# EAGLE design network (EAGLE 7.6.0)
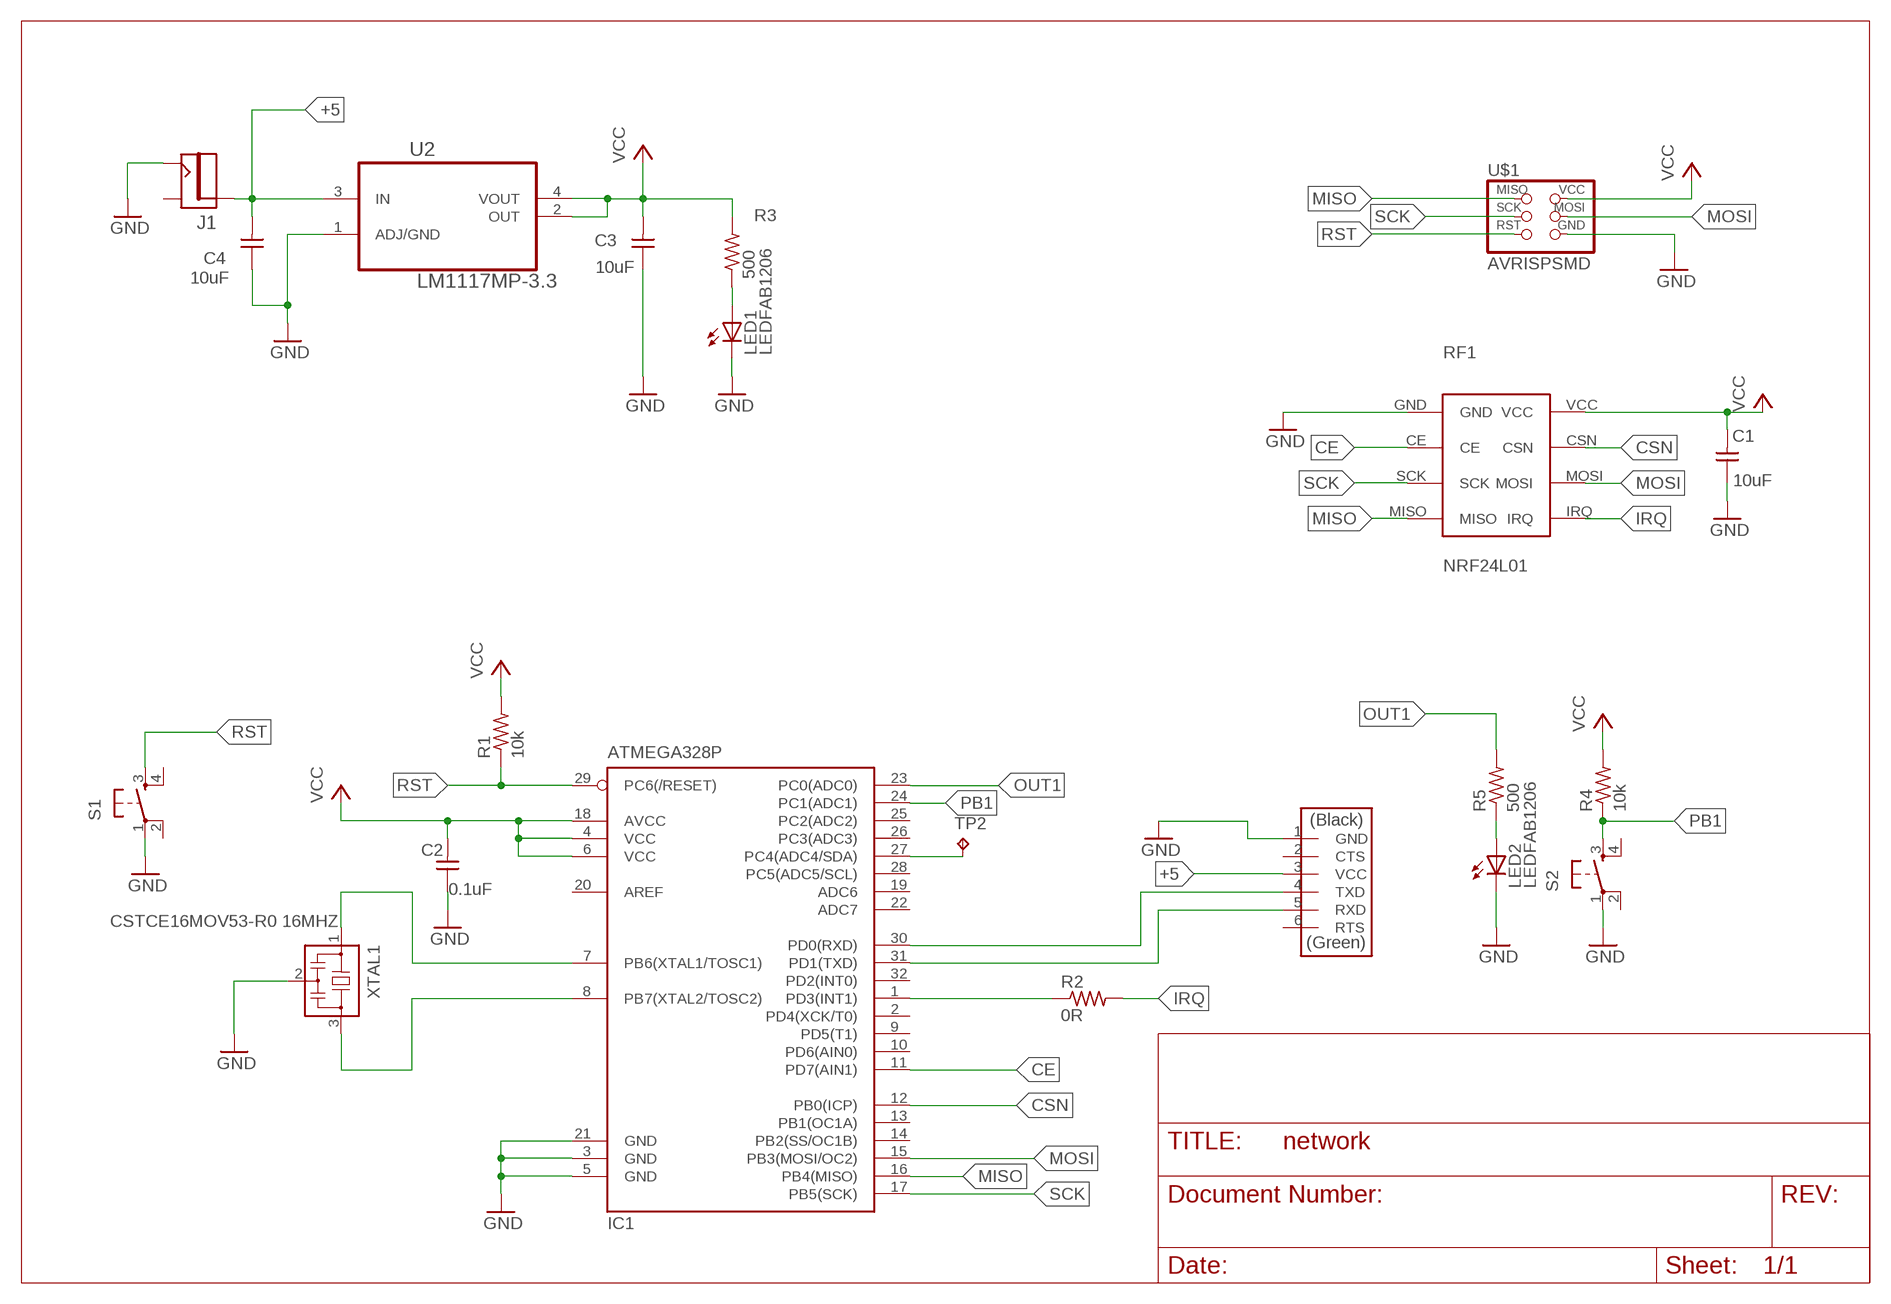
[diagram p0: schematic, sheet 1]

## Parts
C1  10uF  CAP-UNPOLARIZEDFAB  [C1206FAB]
C2  0.1uF  CAP-UNPOLARIZEDFAB  [C1206FAB]
C3  10uF  CAP-UNPOLARIZEDFAB  [C1206FAB]
C4  10uF  CAP-UNPOLARIZEDFAB  [C1206FAB]
IC1  ATMEGA328P  ATMEGA88-THIN  [TQFP32-08THIN]
J1  JACK2.1MM  [JACK_2.1MM]
LED1  LEDFAB1206  [LED1206FAB]
LED2  LEDFAB1206  [LED1206FAB]
R1  10k  RES-US1206FAB  [R1206FAB]
R2  0R  RES-US1206FAB  [R1206FAB]
R3  500  RES-US1206FAB  [R1206FAB]
R4  10k  RES-US1206FAB  [R1206FAB]
R5  500  RES-US1206FAB  [R1206FAB]
RF1  NRF24L01  [NRF24L01]
S1  6MM_SWITCH6MM_SWITCH  [6MM_SWITCH]
S2  6MM_SWITCH6MM_SWITCH  [6MM_SWITCH]
TP2  TPB1,27  [B1,27]
U2  LM1117MP-3.3  [SOT230P696X180-4N]
U$1  AVRISPSMD  [2X03SMD]
U$3  FTDI-SMD-HEADER  [1X06SMD]
XTAL1  CSTCE16MOV53-R0 16MHZ  RESONATOR  [EFOBM]

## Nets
+5: C4.2 J1.PIN U2.3(IN) U$3.3(VCC)
CE: IC1.11(PD7(AIN1)) RF1.CE
CSN: IC1.12(PB0(ICP)) RF1.CSN
GND: C1.1 C2.1 C3.1 C4.1 IC1.3(GND) IC1.5(GND) IC1.21(GND) J1.CONTACT LED1.2(C) LED2.2(C) RF1.GND S1.1(P) S2.1(P) U2.1(ADJ/GND) U$1.6(GND) U$3.1(GND) XTAL1.2
IRQ: R2.2 RF1.IRQ
MISO: IC1.16(PB4(MISO)) RF1.MISO U$1.1(MISO)
MOSI: IC1.15(PB3(MOSI/OC2)) RF1.MOSI U$1.4(MOSI)
N$1: IC1.7(PB6(XTAL1/TOSC1)) XTAL1.1
N$2: IC1.8(PB7(XTAL2/TOSC2)) XTAL1.3
N$3: IC1.30(PD0(RXD)) U$3.4(TXD)
N$4: IC1.31(PD1(TXD)) U$3.5(RXD)
N$6: LED1.1(A) R3.1
N$7: LED2.1(A) R5.1
N$8: IC1.27(PC4(ADC4/SDA)) TP2.TP
N$11: IC1.1(PD3(INT1)) R2.1
OUT1: IC1.23(PC0(ADC0)) R5.2
PB1: IC1.24(PC1(ADC1)) R4.1 S2.3(S)
RST: IC1.29(PC6(/RESET)) R1.1 S1.3(S) U$1.5(RST)
SCK: IC1.17(PB5(SCK)) RF1.SCK U$1.3(SCK)
VCC: C1.2 C2.2 C3.2 IC1.4(VCC) IC1.6(VCC) IC1.18(AVCC) R1.2 R3.2 R4.2 RF1.VCC U2.2(OUT) U2.4(VOUT) U$1.2(VCC)
Unconnected: IC1.2(PD4(XCK/T0)) IC1.9(PD5(T1)) IC1.10(PD6(AIN0)) IC1.13(PB1(OC1A)) IC1.14(PB2(SS/OC1B)) IC1.19(ADC6) IC1.20(AREF) IC1.22(ADC7) IC1.25(PC2(ADC2)) IC1.26(PC3(ADC3)) IC1.28(PC5(ADC5/SCL)) IC1.32(PD2(INT0)) J1.SHUNT S1.2(P1) S1.4(S1) S2.2(P1) S2.4(S1) U$3.2(CTS) U$3.6(RTS)

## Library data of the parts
C1-C4 = fab:CAP-UNPOLARIZED
IC1 = fab:ATMEGA88-THIN
J1 = fab:JACK
LED1 LED2 = fab:LED: LED
R1-R5 = fab:RES-US: Resistor (US Symbol)
RF1 = bs-fablab:NRF24L01
S1 S2 = fab:6MM_SWITCH: OMRON SWITCH
TP2 = testpad:TP: Test pad
U2 = bs-fablab:LM1117MP-3.3: Linear regulators; MPN: LM1117MP-3.3; OC_FARNELL: 9778195; OC_NEWARK: 41K3470; PACKAGE: SOT223-3; SUPPLIER: NationalSemiconductor
U$1 = fab:AVRISP
U$3 = fab:FTDI-SMD-HEADER
XTAL1 = fab:RESONATOR

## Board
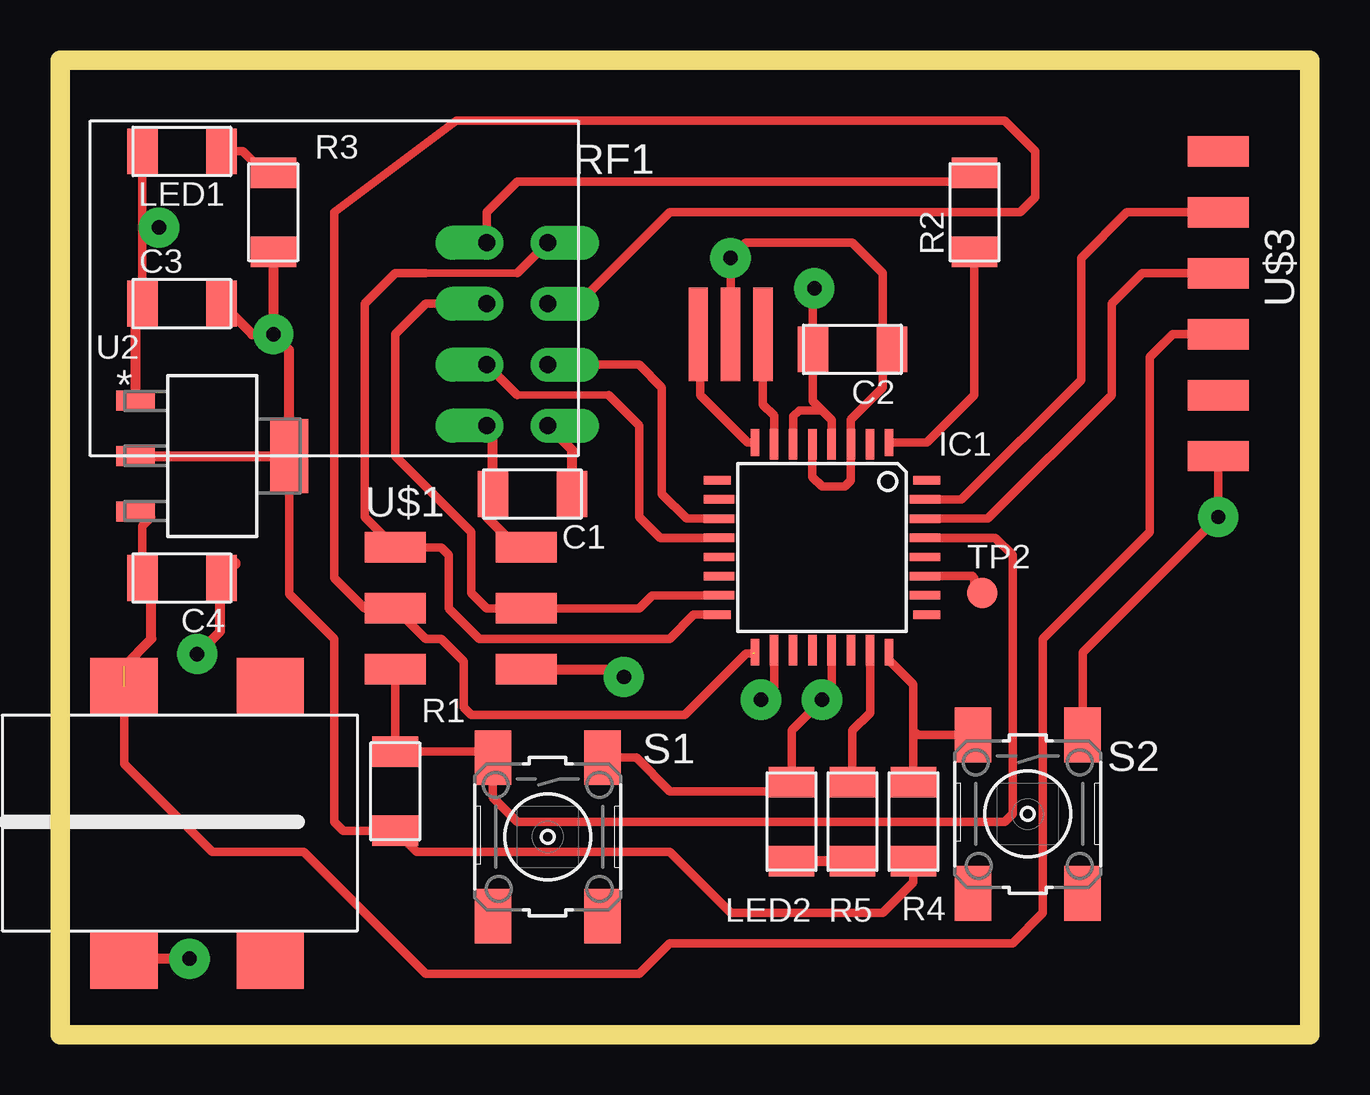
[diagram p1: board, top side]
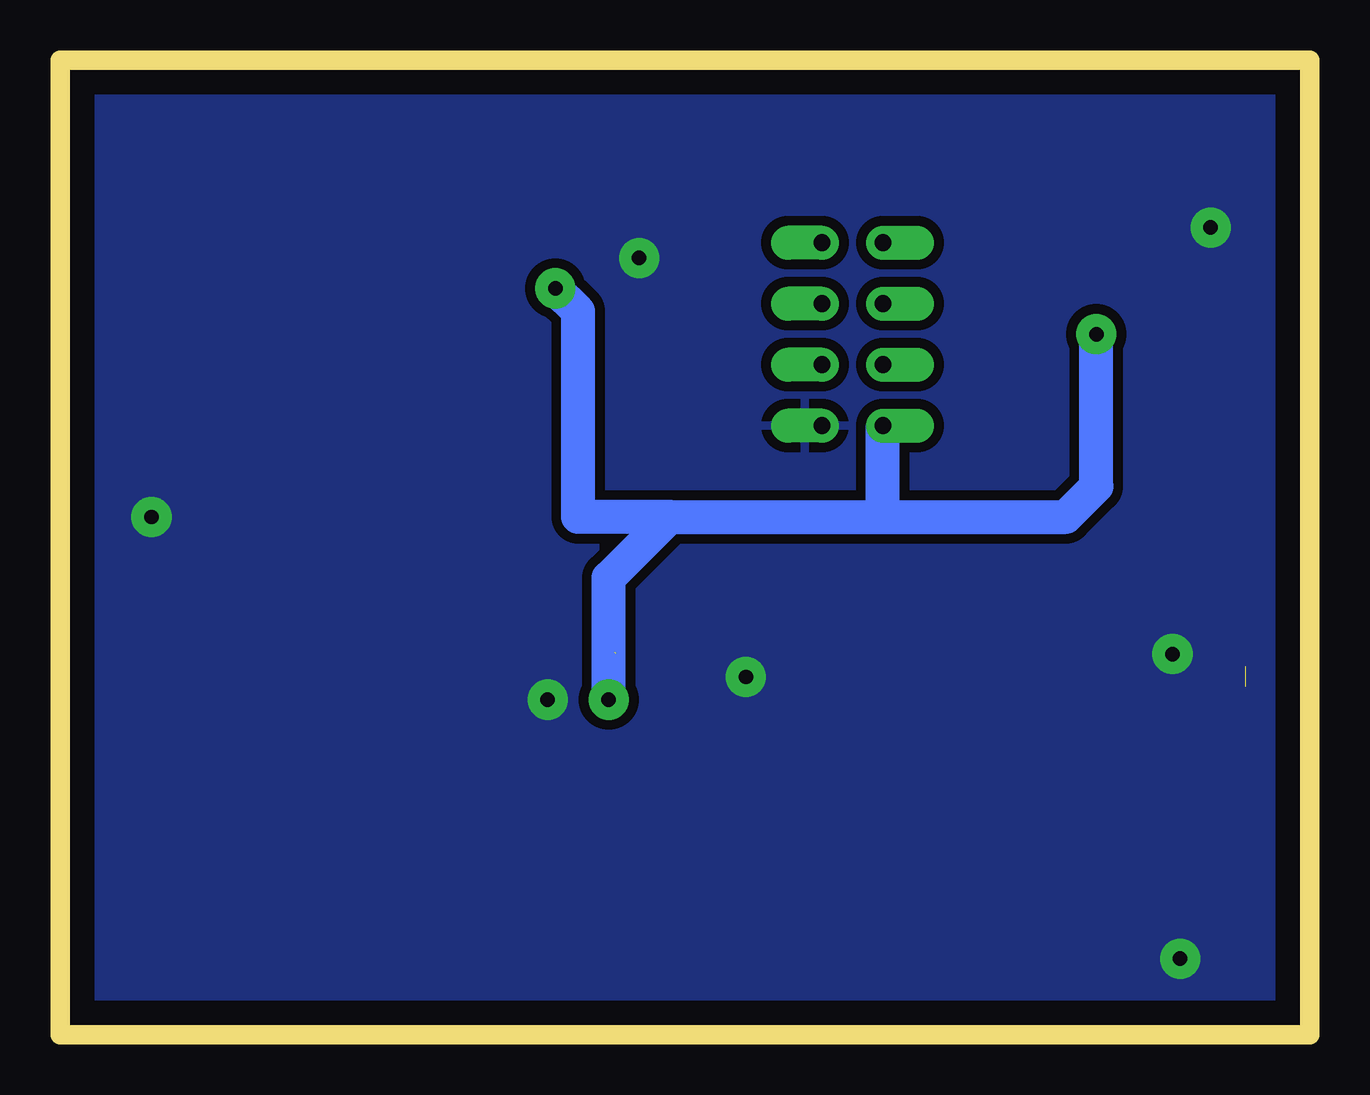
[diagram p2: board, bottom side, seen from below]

Size 52.07 x 40.64 mm. Coordinates in mm from the lower left corner, seen from the top.
Outline: 0,0 52.06,0 52.06,40.63 0,40.63 0,0
Outline: 0,0 0,40.64 52.07,40.64 52.07,0 0,0
Copper layers (1*16): Top 0.035mm / dielectric 1.5mm / Bottom 0.035mm
Design rules "default *": minimum track width 10mil, minimum drill 24mil, track to track 16mil, track to pad 16mil, pad to pad 16mil, via to via 16mil, smd to smd 8mil, copper to edge 40mil, drill to drill 8mil, minimum pad ring 10mil, minimum via ring 8mil, stop-mask expansion 4mil, vias tented up to drill 0mil, thermal gap 16mil

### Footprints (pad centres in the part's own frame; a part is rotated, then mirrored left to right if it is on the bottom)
C1206FAB = smd 1.27 x 1.905: 1 -1.651,0; 2 1.651,0
TQFP32-08THIN = smd 1.118 x 0.356: 1 -4.369,2.8; 8 -4.369,-2.8; 17 4.369,-2.8; 24 4.369,2.8 | smd 1.27 x 0.356: 2 -4.293,2; 3 -4.293,1.2; 4 -4.293,0.4; 5 -4.293,-0.4; 6 -4.293,-1.2; 7 -4.293,-2; 18 4.293,-2; 19 4.293,-1.2; 20 4.293,-0.4; 21 4.293,0.4; 22 4.293,1.2; 23 4.293,2 | smd 0.356 x 1.118: 9 -2.8,-4.369; 16 2.8,-4.369; 25 2.8,4.369; 32 -2.8,4.369 | smd 0.356 x 1.27: 10 -2,-4.293; 14 1.2,-4.293; 15 2,-4.293; 26 2,4.293; 27 1.2,4.293; 31 -2,4.293 | smd 0.35 x 1.27: 11 -1.2,-4.293; 12 -0.4,-4.293; 13 0.4,-4.293; 28 0.4,4.293; 29 -0.4,4.293; 30 -1.2,4.293
JACK_2.1MM = smd 2.388 x 2.794: CONTACT 5.766,-2.413; PIN -5.639,-2.413; PIN1 -5.639,3.683; SHUNT 5.766,3.683
LED1206FAB = smd 1.27 x 1.905: 1 -1.651,0; 2 1.651,0
R1206FAB = smd 1.27 x 1.905: 1 -1.651,0; 2 1.651,0
NRF24L01 = drill 0.7 pad 1.422 offset: CE 1.27,-3.81; CSN 3.81,-3.81; GND 1.27,-1.27; IRQ 3.81,-8.89; MISO 1.27,-8.89; MOSI 3.81,-6.35; SCK 1.27,-6.35; VCC 3.81,-1.27
6MM_SWITCH = smd 2.286 x 1.524: 1 -3.302,2.286; 2 3.302,2.286; 3 -3.302,-2.286; 4 3.302,-2.286
B1,27 = smd 1.27 x 1.27: TP 0,0
SOT230P696X180-4N = smd 1.6 x 0.838: 1 -3.2,2.311; 2 -3.2,0; 3 -3.2,-2.311 | smd 1.6 x 3.099: 4 3.2,0
2X03SMD = smd 2.54 x 1.27: 1 -2.54,2.54; 2 2.92,2.54; 3 -2.54,0; 4 2.92,0; 5 -2.54,-2.54; 6 2.92,-2.54
1X06SMD = smd 2.54 x 1.27: 1 0,6.35; 2 0,3.81; 3 0,1.27; 4 0,-1.27; 5 0,-3.81; 6 0,-6.35
EFOBM = smd 0.8 x 3.9: 1 -1.35,0; 2 0,0; 3 1.35,0

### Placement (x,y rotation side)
C1  19.68,22.54 180 top
C2  33.02,28.57 180 top
C3  5.08,30.48 0 top
C4  5.08,19.05 180 top
IC1  31.75,20.32 270 top
J1  5.08,8.89 270 top
LED1  5.08,36.83 180 top
LED2  30.48,8.89 90 top
R1  13.97,10.16 270 top
R2  38.1,34.29 90 top
R3  8.89,34.29 270 top
R4  35.56,8.89 270 top
R5  33.02,8.89 90 top
RF1  21.59,24.13 180 top
S1  20.32,8.26 270 top
S2  40.32,9.21 270 top
TP2  38.42,18.41 0 top
U2  6.35,24.13 0 top
U$1  16.51,17.78 0 top
U$3  48.26,30.48 180 top
XTAL1  27.94,29.21 180 top

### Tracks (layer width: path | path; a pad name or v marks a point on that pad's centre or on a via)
+5  (1 unrouted)
  Top 0.356: C4.2 3.43,21.21 3.81,21.59 3.38,21.59 U2.3 | U$3.3 46.35,29.21 45.4,28.26 45.4,20.95 40.96,16.51 40.96,5.08 39.69,3.81 25.4,3.81 24.13,2.54 15.24,2.54 10.16,7.62 6.35,7.62 2.67,11.3 J1.PIN
  Top 0.406: 2.67,15.37 3.81,16.51 3.81,18.67 C4.2
CE
  Top 0.356: IC1.11 26.11,21.52 25.08,22.54 25.08,26.99 24.13,27.94 RF1.CE
CSN
  Top 0.305: 19.05,26.67 22.86,26.67
  Top 0.356: RF1.CSN 19.05,26.67 | 22.86,26.67 24.13,25.4 24.13,21.59 25,20.72 IC1.12
GND  (via drill 0.6 pad 1.68)
  Top 0.356: IC1.21 32.15,14.37 v31.75,13.97 30.48,12.7 LED2.2 30.1,10.16 25.4,10.16 24,11.56 S1.1 | IC1.5 31.35,23.26 31.75,22.86 32.7,22.86 32.95,23.11 IC1.3 32.95,25.65 34.29,26.99 34.29,28.19 C2.1 34.29,28.96 34.29,31.75 33.02,33.02 28.57,33.02 v27.94,32.38 XTAL1.2 | C3.1 3.43,33.66 | 3.43,33.66 LED1.2 | v4.13,33.66 3.43,33.66 | U$3.1 v48.26,21.59 42.61,15.94 S2.1
  Top 0.406: U2.1 3.15,30.2 C3.1 | C1.1 21.34,24.38 RF1.GND | v5.71,15.87 6.67,16.83 6.67,19.05 7.3,19.68 7.3,19.62 C4.1 | U$1.6 23.18,15.24 v23.5,14.92 | v5.4,3.17 2.67,3.17 J1.CONTACT
  pour Bottom: 0,40.64 52.07,40.64 52.07,0 0,0
IRQ
  Top 0.356: RF1.IRQ 17.78,34.29 19.05,35.56 37.72,35.56 R2.2
MISO
  Top 0.305: 19.05,31.75 15.24,31.75 14.61,31.75
  Top 0.356: IC1.16 26.41,17.52 25.4,16.51 17.46,16.51 16.19,17.78 16.19,20 15.88,20.32 U$1.1 | 13.02,20.32 U$1.1 | RF1.MISO 19.05,31.75 | U$1.1 12.7,21.59 12.7,30.48 13.97,31.75 15.24,31.75
MOSI
  Top 0.356: IC1.15 24.67,18.32 24.13,17.78 U$1.4 17.78,17.78 17.14,18.41 17.14,20.95 13.97,24.13 13.97,29.21 15.24,30.48 RF1.MOSI
N$1
  Top 0.356: IC1.7 29.75,25.81 29.29,26.27 XTAL1.1
N$2
  Top 0.356: IC1.8 28.65,24.69 26.67,26.67 26.67,29.13 XTAL1.3
N$3
  Top 0.356: IC1.30 38.66,21.52 43.81,26.67 43.81,30.48 45.09,31.75 U$3.4
N$4
  Top 0.356: IC1.31 37.56,22.32 42.55,27.3 42.55,32.38 44.45,34.29 U$3.5
N$6
  Top 0.356: R3.1 8.51,35.94 7.62,36.83 LED1.1
N$7
  Top 0.406: R5.1 LED2.1
N$8
  Top 0.356: IC1.27 38.03,19.12 38.1,19.05 38.1,18.73 TP2.TP
N$11
  Top 0.356: IC1.1 36.12,24.69 38.1,26.67 R2.1
OUT1
  Top 0.356: IC1.23 33.75,13.43 33.02,12.7 R5.2
PB1
  Top 0.356: IC1.24 34.55,15.62 35.56,14.6 35.56,12.7 | R4.1 35.56,12.7 | S2.3 35.75,12.51 35.56,12.7
RST
  Top 0.356: U$1.5 R1.1 17.78,11.81 S1.3 18.03,9.91 19.05,8.89 39.37,8.89 39.69,9.21 39.69,20 38.97,20.72 IC1.29
SCK  (1 unrouted)
  Top 0.356: 28.89,15.89 28.59,15.89 26.04,13.33 17.14,13.33 16.83,13.65 16.83,15.56 15.88,16.51 15.24,16.51 U$1.3 12.7,17.78 11.43,19.05 11.43,34.29 16.51,38.1 39.37,38.1 40.64,36.83 40.64,34.92 40.01,34.29 25.4,34.29 21.59,30.48 RF1.SCK
VCC  (via drill 0.6 pad 1.68)
  Top 0.356: IC1.18 29.75,14.51 v29.21,13.97 | IC1.6 30.55,25.79 30.8,26.03 31.75,26.03 | 31.75,26.03 32.15,25.63 IC1.4 | 31.75,26.03 31.37,26.42 C2.2 31.37,31.05 v31.43,31.11 | U2.4 9.55,18.39 11.43,16.51 11.43,8.89 11.81,8.51 R1.2 14.86,7.62 25.4,7.62 27.94,5.08 34.29,5.08 35.56,6.35 R4.2
  Top 0.406: U2.2 U2.4 9.55,28.55 v8.89,29.21 | RF1.VCC 18.03,25.15 C1.2 17.78,22.29 17.78,21.59 19.05,20.32 U$1.2 | v8.89,29.21 8,29.21 C3.2 | R3.2 v8.89,29.21
  Bottom 1.422: v29.21,13.97 29.21,19.05 26.67,21.59 | 26.67,21.59 17.78,21.59 | 17.78,21.59 RF1.VCC | 17.78,21.59 10.16,21.59 8.89,22.86 v8.89,29.21 | 26.67,21.59 30.48,21.59 30.48,30.16 v31.43,31.11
